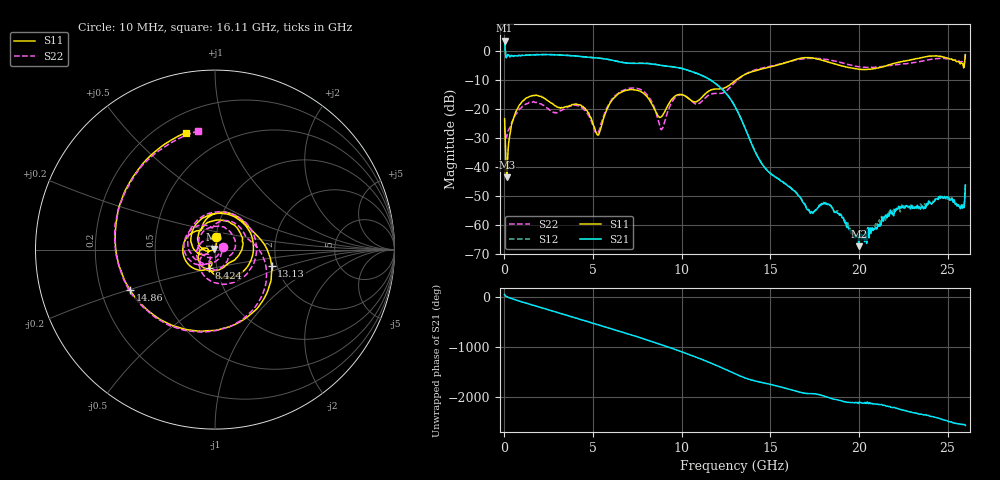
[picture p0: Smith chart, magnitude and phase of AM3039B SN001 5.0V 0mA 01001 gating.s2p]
!Agilent Technologies,E8364B,MY43040894,A.07.50.67
!Agilent E8364B: A.07.50.67
!Date: Tuesday, June 28, 2016 08:05:22
!Correction: S11(Full 2 Port(1,2))
!S21(Full 2 Port(1,2))
!S12(Full 2 Port(1,2))
!S22(Full 2 Port(1,2))
!S2P File: Measurements: S11, S21, S12, S22:
# Hz S  dB  R 50
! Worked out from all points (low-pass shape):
!   1601 points, 10 MHz to 26 GHz, reference 50 ohm
!   highest |S21| = 3.62 dB at 10 MHz (marker M1); lowest = -67.3 dB at 19.99 GHz (marker M2)
!   |S21| within 3 dB of the highest: start of sweep to 44.42 MHz
!   lowest |S11| = -43.5 dB at 139.9 MHz (marker M3), VSWR 1.01, Z = 49.4 + j0.332 ohm
!   |S11| at or under -10 dB: start of sweep to 13.06 GHz
!   |S22| runs from -29.8 to -0.8 dB; largest |S21 - S12| = 0.024
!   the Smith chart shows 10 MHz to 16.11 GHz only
!   S11 on the Smith chart (normalised r, x): 10 MHz: 1.00, +0.14; 8.424 GHz: 0.92, -0.19; 13.13 GHz: 1.87, -0.39; 14.86 GHz: 0.33, -0.20; 16.11 GHz: 0.31, +0.74
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1e7  -23.29 87.0  3.62 40.6  3.68 41.4  -26.36 17.5
1.3995e8  -43.55 149.7  -1.69 -1.7  -1.64 -1.6  -29.17 -62.4
8.221875e8  -18.75 147.3  -1.53 -87.7  -1.46 -87.6  -20.23 166.1
1.618131e9  -15.26 66.3  -1.27 -171.8  -1.22 -171.7  -17.45 71.7
2.495294e9  -17.28 -13.0  -1.22 96.5  -1.15 96.6  -20.00 -11.0
3.307481e9  -19.47 -55.1  -1.40 11.0  -1.33 11.1  -20.11 -54.5
4.347081e9  -18.88 -137.3  -1.89 -99.7  -1.86 -99.6  -19.44 -163.6
5.809019e9  -19.71 -172.3  -2.82 101.3  -2.77 101.6  -19.21 -142.1
6.816131e9  -13.59 71.1  -4.05 -6.6  -4.00 -6.3  -13.23 68.0
8.424262e9  -19.46 -107.5  -4.51 174.3  -4.45 174.5  -19.01 -141.0
8.684162e9  -22.53 -111.5  -4.76 143.8  -4.70 144.0  -23.94 -154.8
9.804981e9  -14.99 -167.8  -5.72 8.4  -5.65 8.5  -15.26 176.6
1.3005e10  -10.26 -7.0  -19.09 -93.0  -19.04 -93.2  -10.77 -14.8
1.313495e10  -9.65 -16.5  -20.58 -113.3  -20.53 -113.5  -10.02 -24.3
1.485679e10  -5.61 -154.3  -41.40 67.2  -41.32 66.6  -5.40 -164.3
1.610756e10  -3.46 103.8  -46.90 -45.3  -46.88 -45.5  -3.51 98.0
1.734208e10  -2.34 -13.8  -55.37 -131.0  -55.90 -131.3  -2.46 -7.9
1.998981e10  -6.28 128.4  -67.25 52.3  -62.92 45.6  -5.39 139.1
2.167916e10  -4.72 15.9  -56.76 -25.9  -55.56 -26.9  -5.00 22.0
2.312486e10  -2.75 -92.5  -54.27 -149.8  -53.81 -152.1  -3.93 -82.6
2.422943e10  -1.64 177.8  -51.83 129.1  -51.94 129.1  -2.68 -166.6
2.6e10  -1.33 -21.4  -46.20 -40.3  -45.69 -39.1  -0.78 8.0
